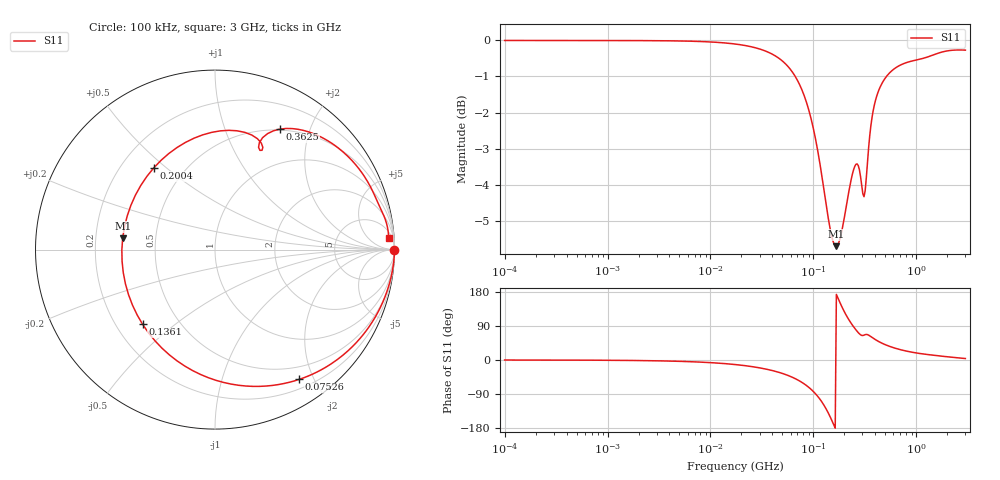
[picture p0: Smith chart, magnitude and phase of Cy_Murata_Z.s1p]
!Murata Part Number: GA242QR7E2102MW01
!X7R ceramic capacitor, package code size 1808, 250 Vac, 1 nF +/-20%, -55°c to 125°c
!Impedance provided by the manufacturer
# HZ Z MA R 50
!Freq.(Hz) Z11(Mag) Z11(Phase)
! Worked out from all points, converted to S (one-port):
!   401 points, 100 kHz to 3 GHz, reference 50 ohm
!   lowest |S11| = -5.7 dB at 167.3 MHz (marker M1), VSWR 3.15, Z = 15.9 + j2.73 ohm
!   |S11| at or under -10 dB: nowhere
!   S11 on the Smith chart (normalised r, x): 100 kHz: open; 75.26 MHz: 0.32, -1.80; 136.1 MHz: 0.31, -0.39; 200.4 MHz: 0.34, +0.45; 362.5 MHz: 0.49, +1.56; 3 GHz: 11, +24
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100000  1575 -88.2
362777.3  441.8 -89.0
1316074  123.1 -89.0
4774418  34.25 -88.5
1.732051e7  9.539 -86.9
3.752708e7  4.3 -84.9
4.982709e7  3.125 -83.6
6.283488e7  2.346 -81.9
7.525761e7  1.826 -79.9
9.013636e7  1.365 -76.8
1.0521e8  1.009 -72.2
1.196798e8  0.737 -65.3
1.361397e8  0.4969 -51.4
1.509232e8  0.3547 -28.1
1.673121e8  0.323 9.7
1.807614e8  0.3936 34.5
2.003904e8  0.5651 53.4
2.279507e8  0.8444 64.2
2.52704e8  1.112 67.4
2.801453e8  1.407 65.5
3.105665e8  1.468 60.3
3.355313e8  1.464 66.6
3.625028e8  1.639 72.7
4.231245e8  2.115 77.6
5.067781e8  2.734 79.6
8.269535e8  4.906 79.8
1.701687e9  10.57 78.1
3e9  26.72 65.5
